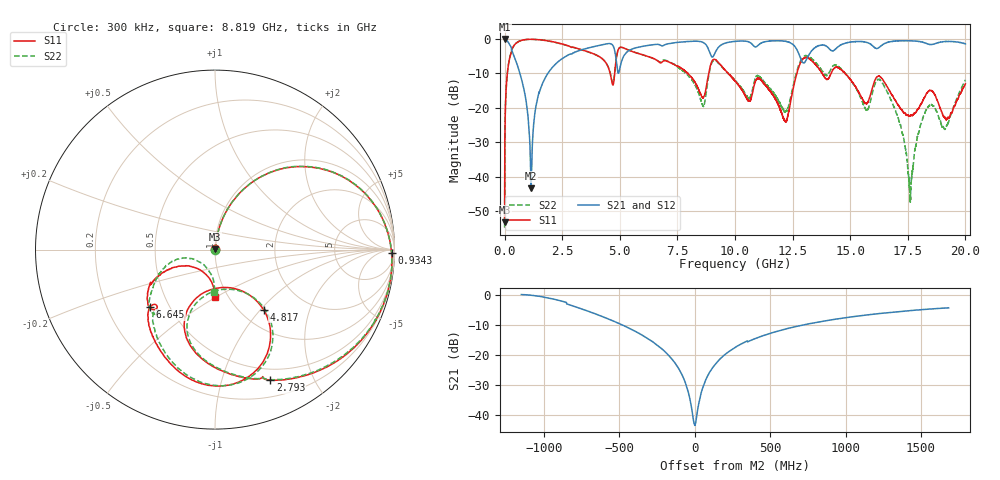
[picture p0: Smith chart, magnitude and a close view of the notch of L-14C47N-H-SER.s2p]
!{L-14C47N}
!Johanson Technology Inc.
!www.johansontechnology.com
!Test Board Conditions:
!Substrate Type  RO4350B
!Substrate Thickness  20 mil
!Substrate Dk  3.66
!TL Type: GCPW
!TL Trace Width  36 mil
!TL Gap  12 mil
!Electrode orientation  Horizontal
!DUT TOPOLOGY	SERIES
!Mounting Pad LxW  26x36 mil
! Created Sun Jun 20 13:06:00 2021
# hz S ma R 50
! 2 Port Network Data from SP1.SP block
! freq  magS11  angS11  magS21  angS21  magS12  angS12  magS22  angS22
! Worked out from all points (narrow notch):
!   20001 points, 300 kHz to 20 GHz, reference 50 ohm
!   highest |S21| = -0.01 dB at 1.3 MHz (marker M1); lowest = -43.4 dB at 1.15 GHz (marker M2)
!   notch at M2: 41.8 dB deep, 281 MHz wide at half that depth
!   lowest |S11| = -53.3 dB at 300 kHz (marker M3), VSWR 1.00, Z = 50.2 + j0.0934 ohm
!   |S11| at or under -10 dB: 7.953 GHz to 8.857 GHz (903.6 MHz wide, 10.7 % of centre); 9.707 GHz to 12.68 GHz (2.975 GHz wide, 26.6 % of centre); 14.78 GHz to end of sweep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
!   |S22| runs from -54.9 to -0.1 dB; largest |S21 - S12| = 0.013
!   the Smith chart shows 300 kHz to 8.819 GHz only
!   S11 on the Smith chart (normalised r, x): 300 kHz: 1.00, +0.00; 934.3 MHz: 47, -63; 2.793 GHz: 0.38, -1.44; 4.817 GHz: 1.27, -1.04; 6.645 GHz: 0.39, -0.33; 8.819 GHz: 0.87, -0.50
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300000  0.002167 25.4  0.9988 -0.1  0.9969 -0.0  0.001804 7.6
1300000  0.00369 75.3  0.9989 -0.2  0.9987 -0.3  0.003865 73.9
1.053e8  0.2847 70.0  0.9455 -17.6  0.9463 -17.5  0.2858 69.9
2.033e8  0.4985 56.5  0.8516 -31.8  0.8521 -31.7  0.4999 56.5
9.343e8  0.9848 -1.2  0.1245 -87.6  0.1245 -87.7  0.9838 -1.1
1.1503e9  0.9918 -10.6  0.00678 -11.5  0.006833 -10.8  0.9913 -10.5
1.5813e9  0.9726 -26.3  0.1987 62.0  0.1994 61.9  0.9704 -26.2
2.7933e9  0.7892 -67.0  0.5931 22.0  0.5937 21.9  0.7879 -66.9
3.3343e9  0.7012 -82.6  0.6958 6.3  0.6971 6.3  0.6974 -82.5
4.8173e9  0.4298 -51.0  0.5749 -66.2  0.5746 -66.1  0.4383 -50.2
5.0853e9  0.7582 -91.7  0.4844 -15.9  0.4849 -15.7  0.7572 -89.8
6.6453e9  0.4815 -138.6  0.8375 -51.0  0.84 -50.9  0.4831 -134.4
6.6673e9  0.4744 -138.6  0.8365 -51.6  0.8382 -51.5  0.4782 -134.4
8.8193e9  0.2684 -89.9  0.7508 -103.9  0.7498 -104.0  0.2411 -91.0
1.00003e10  0.2462 -176.6  0.9248 -100.3  0.9264 -100.3  0.2502 176.5
1.21873e10  0.06437 -158.5  0.9267 -142.7  0.9294 -142.7  0.08651 -168.9
1.33343e10  0.4826 162.5  0.6777 -130.3  0.6746 -130.5  0.5162 162.5
1.66673e10  0.1853 117.0  0.904 178.3  0.9051 178.7  0.1576 101.3
1.76053e10  0.07614 145.6  0.9439 157.9  0.9447 157.9  0.004596 -23.7
1.83213e10  0.1635 162.1  0.8597 144.1  0.8583 144.1  0.09605 -172.5
1.91393e10  0.06931 142.0  0.9195 134.7  0.9213 134.8  0.05074 151.3
2e10  0.223 178.2  0.85 112.0  0.8414 111.8  0.2543 172.8
